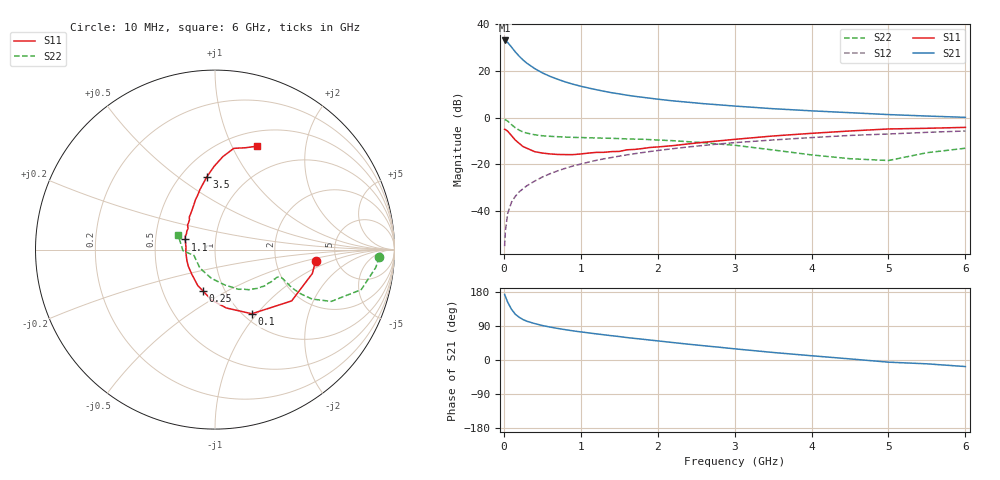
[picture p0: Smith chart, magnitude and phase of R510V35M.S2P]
! SIEMENS Small Signal Semiconductors
! BFR183
! Si NPN RF Bipolar Junction Transistor in SOT23
! VCE = 10 V  IC = 35 mA
! Common Emitter S-Parameters:  May  1996
# GHz  S  MA  R  50
!  f  S11  S21  S12  S22
! GHz  MAG  ANG  MAG  ANG  MAG  ANG  MAG  ANG
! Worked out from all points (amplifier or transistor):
!   36 points, 10 MHz to 6 GHz, reference 50 ohm
!   highest |S21| = 33.0 dB at 10 MHz (marker M1)
!   |S21| within 3 dB of that: start of sweep to 103.7 MHz
!   unconditionally stable (mu >= 1): 486.3 MHz to 2.548 GHz
!   at 250 MHz: K = 0.87, MSG = 27.5 dB, |S12| = -30.3 dB
!   at 1.4 GHz: K = 1.05, MAG = 12.5 dB, |S12| = -17.0 dB
!   at 6 GHz: K = 0.90, MSG = 2.9 dB, |S12| = -5.7 dB
!   S11 on the Smith chart (normalised r, x): 10 MHz: 3.45, -0.66; 100 MHz: 1.09, -0.94; 250 MHz: 0.79, -0.39; 1.1 GHz: 0.71, +0.08; 3.5 GHz: 0.66, +0.64; 6 GHz: 0.67, +1.25
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0.01  0.564 -6.6  44.58 173.2  0.0018 65.9  0.9159 -2.6
0.02  0.5585 -13.8  43.69 167.6  0.0038 80.3  0.9017 -6.3
0.05  0.5139 -33.8  40.4 152.6  0.009 73.4  0.8448 -15.3
0.1  0.4122 -60.1  32.13 133.6  0.0157 69.6  0.7094 -24.0
0.15  0.3315 -79.0  25.27 120.6  0.021 67.8  0.6077 -27.0
0.2  0.2818 -93.9  20.52 112.6  0.026 69.3  0.5404 -27.3
0.25  0.2412 -105.7  17.03 106.6  0.0304 69.9  0.4944 -26.7
0.3  0.2219 -115.7  14.53 102.3  0.0352 71.0  0.4673 -26.0
0.4  0.188 -133.7  11.22 96.2  0.0441 72.2  0.4317 -24.3
0.5  0.1755 -147.7  9.06 91.0  0.0539 72.8  0.4105 -23.2
0.6  0.1682 -158.5  7.638 86.9  0.0634 72.7  0.3998 -23.0
0.7  0.1637 -167.8  6.603 83.3  0.0732 72.5  0.3921 -23.2
0.8  0.1626 -177.1  5.797 80.0  0.083 71.5  0.3848 -23.4
0.9  0.1624 175.3  5.175 76.9  0.0929 71.1  0.3796 -23.9
1.1  0.1752 161.2  4.302 71.6  0.1123 70.0  0.3724 -25.9
1.3  0.1818 151.0  3.668 66.6  0.132 67.9  0.3646 -28.0
1.6  0.2058 138.1  3.02 59.2  0.1605 64.9  0.3515 -32.2
2.2  0.2528 120.7  2.283 46.0  0.2178 58.4  0.3224 -42.0
3.5  0.4061 96.6  1.554 19.9  0.3343 41.9  0.2041 -74.6
4.5  0.5196 85.2  1.277 2.9  0.4175 29.5  0.1328 -129.2
5.5  0.593 73.2  1.083 -10.1  0.4858 18.3  0.1785 -177.9
6  0.6207 68.1  1.016 -17.3  0.519 11.0  0.2223 158.1
